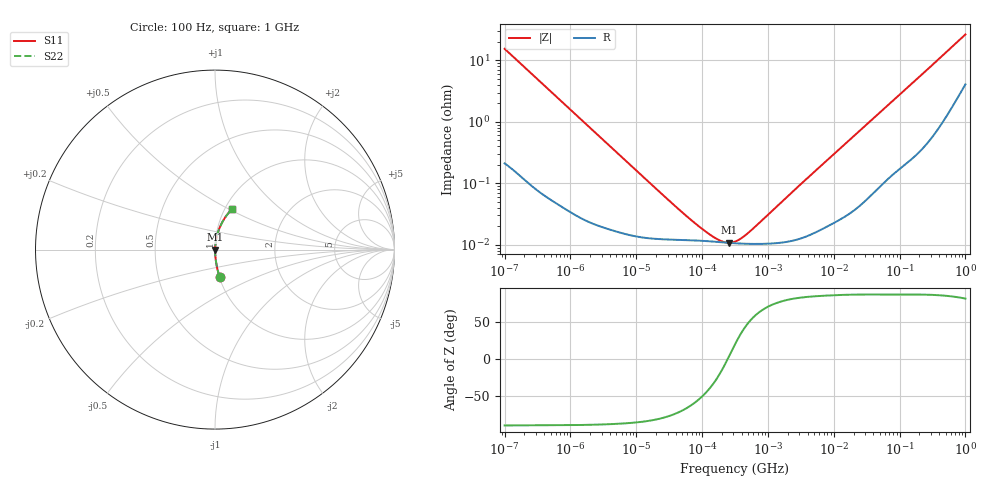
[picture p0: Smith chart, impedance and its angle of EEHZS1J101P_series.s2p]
!  *** S-Parameter ***
!  Copyright (C) Panasonic Industry
!  Conductive Polymer Hybrid Aluminum Electrolytic Capacitors
!  Parts No. EEHZS1J101P
!  Connection Mode : Series
!  1  o---||---o  2
!  GND o--------o GND
!  Conditions : Temperature = 20 degC , DC Bias = 0 V
! Frequency Range : 100Hz  -  1GHz  [ 401 Steps ]
# Hz S RI R 50
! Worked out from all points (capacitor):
!   401 points, 100 Hz to 1 GHz, reference 50 ohm
!   read as one part in series: C = 103 uF near 108.4 Hz
!   lowest |Z| = 10.7 mohm at 258.5 kHz (marker M1)
!   series resonance near 245 kHz, so ESL is about 4.1 nH
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100  0.0253 -0.1504  0.9747 0.1504  0.9747 0.1504  0.0253 -0.1504
108.3927  0.0218 -0.1394  0.9782 0.1394  0.9782 0.1394  0.0218 -0.1394
175.7924  0.00903 -0.0876  0.991 0.0876  0.991 0.0876  0.00903 -0.0876
309.0295  0.00332 -0.0504  0.9967 0.0504  0.9967 0.0504  0.00332 -0.0504
1487.647  0.000379 -0.0106  0.9996 0.0106  0.9996 0.0106  0.000379 -0.0106
22130.95  0.000124 -0.000727  0.9999 0.000727  0.9999 0.000727  0.000124 -0.000727
58210.32  0.000119 -0.000266  0.9999 0.000266  0.9999 0.000266  0.000119 -0.000266
115478.2  0.000115 -0.000114  0.9999 0.000114  0.9999 0.000114  0.000115 -0.000114
153108.7  0.000112 -6.83e-05  0.9999 6.83e-05  0.9999 6.83e-05  0.000112 -6.83e-05
187283.7  0.00011 -3.86e-05  0.9999 3.86e-05  0.9999 3.86e-05  0.00011 -3.86e-05
220039.2  0.000109 -1.54e-05  0.9999 1.54e-05  0.9999 1.54e-05  0.000109 -1.54e-05
258523.5  0.000107 7.8e-06  0.9999 -7.8e-06  0.9999 -7.8e-06  0.000107 7.8e-06
316227.8  0.000106 3.78e-05  0.9999 -3.78e-05  0.9999 -3.78e-05  0.000106 3.78e-05
402717  0.000104 7.67e-05  0.9999 -7.67e-05  0.9999 -7.67e-05  0.000104 7.67e-05
533949.3  0.000103 0.000128  0.9999 -0.000128  0.9999 -0.000128  0.000103 0.000128
4704354  0.000151 0.00142  0.9998 -0.00142  0.9998 -0.00142  0.000151 0.00142
6.99842e7  0.00161 0.0194  0.9984 -0.0194  0.9984 -0.0194  0.00161 0.0194
1.566751e8  0.00431 0.0421  0.9957 -0.0421  0.9957 -0.0421  0.00431 0.0421
2.985383e8  0.0115 0.0786  0.9885 -0.0786  0.9885 -0.0786  0.0115 0.0786
5.922431e8  0.0385 0.1488  0.9615 -0.1488  0.9615 -0.1488  0.0385 0.1488
9.225714e8  0.084 0.2142  0.916 -0.2142  0.916 -0.2142  0.084 0.2142
1e9  0.0962 0.2271  0.9038 -0.2271  0.9038 -0.2271  0.0962 0.2271
